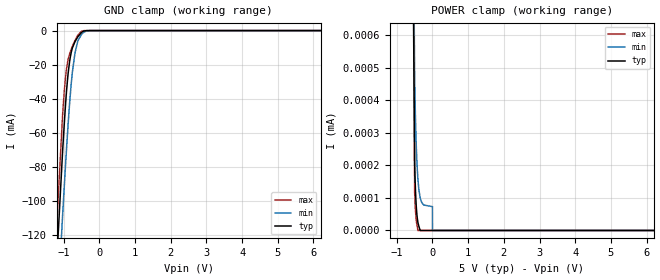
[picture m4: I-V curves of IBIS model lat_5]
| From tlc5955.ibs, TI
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|   lat_5 Model
[Model]   lat_5
Model_type   Input
Vinl = 1.5
Vinh = 3.5
|   typ   min   max
|   (nom PVT)   (fast PVT)   (slow PVT)
C_comp   1.508e-12   1.451e-12   1.577e-12
[Model spec]
|subparameter
Vinl   1.5   1.35   1.65
Vinh   3.5   3.15   3.85
| Where nom  PVT is Nominal Process, 5V, 27C
|   Fast PVT is Strong Process,  5.5V, -40C
|   Slow PVT is Weak Process,   4.5V, 125C
[Voltage Range]   5   4.5   5.5
|Junction Temperature
[Temperature Range]   27   125   -40
[Power Clamp Reference]   5   4.5   5.5
[GND Clamp Reference]   0   0   0
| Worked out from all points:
|   GND clamp passes 1 mA (typ) near -0.50 V on its own axis
|   POWER clamp passes 1 mA (typ) near -2.90 V on its own axis
[GND Clamp]
|   Voltage   I(typ)   I(min)   I(max)
-5V       -1.866A    -1.837A    -1.898A
-1.215V   -143.6mA   -180.1mA   -122.8mA
-1.036V   -73.23mA   -110.9mA   -51.8mA
-979.5mV  -53.55mA   -90.37mA   -34.62mA
-925mV    -36.92mA   -71.33mA   -23.3mA
-833mV    -18.12mA   -42.62mA   -13.66mA
-755mV    -10.15mA   -24.32mA   -9.237mA
-682.5mV  -6.493mA   -13.14mA   -5.774mA
-603.5mV  -3.647mA   -6.114mA   -2.71mA
-484.5mV  -823.3uA   -1.885mA   -282uA
-220.5mV  -668.5nA   -16.11uA   -26nA
10V       0A         0A         0A
[POWER Clamp]
|   Voltage   I(typ)   I(min)   I(max)
-5V       130.2mA    91.47mA    167.3mA
-2.267V   25.46uA    25.66uA    46.7uA
-500mV    207.4nA    472.8nA    118.4nA
-482mV    139.7nA    370.9nA    71.24nA
-459.5mV  83.72nA    277.8nA    36.58nA
-437mV    49.53nA    212.8nA    18.23nA
-410mV    25.9nA     160.7nA    0A
-378.5mV  12.08nA    123.6nA    0A
-302mV    0A         86.34nA    0A
-500uV    0A         73.33nA    0A
-84.44fV  0A         0A         0A
10V       0A         0A         0A
